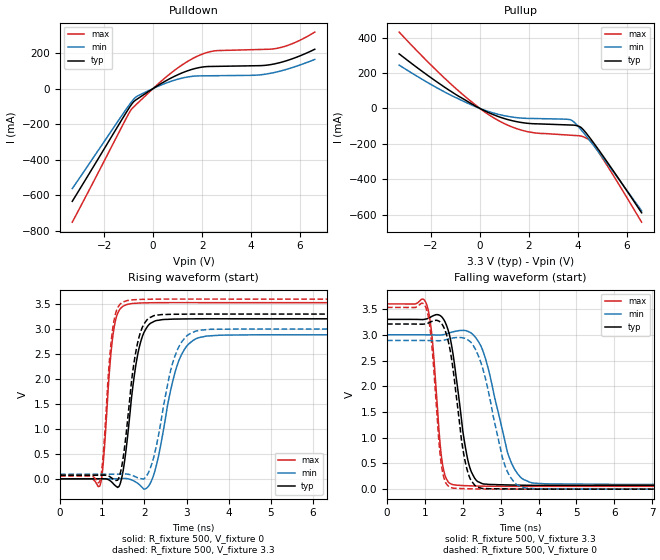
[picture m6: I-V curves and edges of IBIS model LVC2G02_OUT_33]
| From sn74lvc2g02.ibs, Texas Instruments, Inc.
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[Model]   LVC2G02_OUT_33
Model_type  Output
Vref =   0
Rref =   500
Cref =   50p
Vmeas =   1.5
| variable   typ   min   max
C_comp   8.64pF   6.35pF   12.84pF
| C_pullup   8.05pF   6.35pF   9.24pF
| C_pulldown   9.23pF   6.40pF   12.84pF
[Temperature Range]   40   100   -40
| Ambient temperature   25   85   -40
[Voltage range]   3.3   3   3.6
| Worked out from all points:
|   slope of the pulldown table from 0 to 0.495 V, typ, clamps not added: 11.9 ohm
|   slope of the pullup table from 0 to 0.495 V, typ, clamps not added: 15.5 ohm
|   rising waveform, R_fixture 500, V_fixture 0: 20-80 % time 286ps typ, 427ps min, 187ps max; typ from 0 V to 3.21 V
|   falling waveform, R_fixture 500, V_fixture 3.3: 20-80 % time 356ps typ, 555ps min, 219ps max; typ from 3.3 V to 0.073 V
|   rising waveform, R_fixture 500, V_fixture 3.3: 20-80 % time 280ps typ, 420ps min, 183ps max; typ from 0.073 V to 3.3 V
|   falling waveform, R_fixture 500, V_fixture 0: 20-80 % time 339ps typ, 521ps min, 218ps max; typ from 3.21 V to 0 V
[Pulldown]
| LVC2G02_OUT_33
|   Voltage   I(typ)   I(min)   I(max)
-3.3V     -635.3mA   -563.8mA   -752.9mA
-915mV    -95.9mA    -80.92mA   -123mA
-785mV    -73.2mA    -58.7mA    -102.4mA
-620mV    -56.23mA   -40.97mA   -80.72mA
745mV     60.18mA    41.47mA    89mA
1.53V     105.7mA    67.74mA    162.6mA
2.225V    124.1mA    71.95mA    204mA
2.635V    125.2mA    72.54mA    213.9mA
4.185V    128.6mA    75.28mA    219.5mA
5.06V     142.2mA    93.97mA    226.8mA
5.775V    172.4mA    122.4mA    258.2mA
6.6V      221.3mA    163.7mA    318.2mA
[Pullup]
| LVC2G02_OUT_33
|   Voltage   I(typ)   I(min)   I(max)
-3.3V     307.9mA    244.4mA    430.7mA
-2.135V   186.7mA    146.1mA    263.5mA
-1.115V   90.19mA    69.44mA    128.8mA
-75mV     5.506mA    4.131mA    8.007mA
580mV     -36.72mA   -26.83mA   -54.43mA
1.245V    -66.49mA   -46.97mA   -100.7mA
1.91V     -83.07mA   -55.77mA   -129.6mA
3.75V     -93.52mA   -67.34mA   -151.2mA
4.12V     -106.6mA   -118.8mA   -155.3mA
4.56V     -179.1mA   -194.4mA   -190.4mA
5.29V     -320.8mA   -328.1mA   -343.1mA
6.6V      -588.3mA   -577.1mA   -641.1mA
[Ramp]
| LVC2G02_OUT_33
| variable   typ   min   max
dV/dt_r   2.03/3.07E-10   1.86/4.66E-10   2.21/1.97E-10
dV/dt_f   1.99/3.87E-10   1.80/6.07E-10   2.18/2.29E-10
R_load = 500
[Rising Waveform]
| LVC2G02_OUT_33
R_fixture =   500
C_fixture =   0
L_fixture =   0
V_fixture =   0
V_fixture_min = 0
V_fixture_max = 0
|   Time   V(typ)   V(min)   V(max)
0s        260.7nV    -32.83nV   33nV
945ps     1.197mV    -77.12uV   -135.8mV
1.28ns    -115.3mV   346.6uV    3.028V
1.47ns    51.74mV    6.625mV    3.443V
1.685ns   1.556V     -18.46mV   3.509V
1.87ns    2.608V     -109.5mV   3.521V
2.105ns   3.087V     -138.4mV   3.526V
2.815ns   3.201V     2.364V     3.53V
3.47ns    3.206V     2.86V      3.53V
24.99ns   3.205V     2.883V     3.529V
[Falling Waveform]
| LVC2G02_OUT_33
R_fixture =   500
C_fixture =   0
L_fixture =   0
V_fixture =   3.3
V_fixture_min = 3
V_fixture_max = 3.6
|   Time   V(typ)   V(min)   V(max)
0s        3.3V       3V         3.6V
1.04ns    3.309V     2.999V     3.599V
1.19ns    3.36V      2.998V     2.948V
1.455ns   3.338V     2.998V     531.2mV
1.745ns   2.611V     3.058V     85.35mV
2.065ns   828mV      3.082V     67.94mV
2.31ns    216.9mV    2.971V     61.6mV
3.255ns   80.56mV    560mV      54.59mV
3.85ns    74.13mV    118.8mV    54.48mV
24.99ns   72.55mV    91.99mV    54.93mV
[Rising Waveform]
| LVC2G02_OUT_33
R_fixture =   500
C_fixture =   0
L_fixture =   0
V_fixture =   3.3
V_fixture_min = 3
V_fixture_max = 3.6
|   Time   V(typ)   V(min)   V(max)
0s        72.51mV    91.94mV    54.9mV
940ps     73.59mV    91.86mV    -50.2mV
1.26ns    -9.585mV   92.07mV    3.079V
1.435ns   139.9mV    96.69mV    3.508V
1.605ns   1.218V     93.14mV    3.573V
1.805ns   2.586V     34.66mV    3.59V
2.03ns    3.15V      33.14mV    3.597V
2.725ns   3.297V     2.462V     3.601V
3.3ns     3.3V       2.976V     3.601V
24.99ns   3.3V       3V         3.6V
[Falling Waveform]
| LVC2G02_OUT_33
R_fixture =   500
C_fixture =   0
L_fixture =   0
V_fixture =   0
V_fixture_min = 0
V_fixture_max = 0
|   Time   V(typ)   V(min)   V(max)
0s        3.209V     2.89V      3.532V
1.03ns    3.216V     2.889V     3.519V
1.17ns    3.256V     2.888V     2.889V
1.44ns    3.217V     2.888V     442.1mV
1.74ns    2.345V     2.938V     20.13mV
1.995ns   809.6mV    2.941V     10.82mV
2.22ns    167.2mV    2.849V     6.295mV
3.125ns   5.718mV    433.5mV    -297.7uV
3.67ns    1.411mV    19.63mV    -417.9uV
24.99ns   32.74uV    46.73uV    22.01uV
